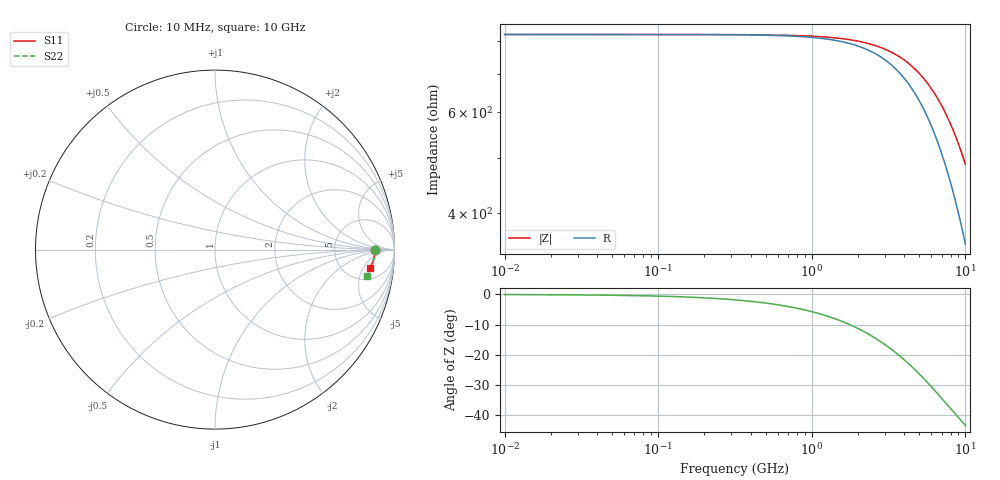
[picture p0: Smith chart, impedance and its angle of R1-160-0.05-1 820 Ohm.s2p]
!version-1
!date-03.2021
# MHz S RI R 50
!Freq ReS11 ImS11 ReS21 ImS21 ReS12 ImS12 ReS22 ImS22
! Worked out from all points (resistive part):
!   501 points, 10 MHz to 10 GHz, reference 50 ohm
!   read as one part in series: R = 820 ohm at 50 MHz
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10  0.8913 -9.71e-05  0.1087 9.47e-05  0.1087 9.47e-05  0.8913 -0.000136
430  0.8913 -0.00418  0.1088 0.00407  0.1088 0.00407  0.8912 -0.00584
850  0.8911 -0.00826  0.1089 0.00806  0.1089 0.00806  0.891 -0.0116
1270  0.8909 -0.0123  0.1092 0.012  0.1092 0.012  0.8907 -0.0173
1690  0.8906 -0.0164  0.1096 0.016  0.1096 0.016  0.8903 -0.023
2090  0.8902 -0.0203  0.11 0.0199  0.11 0.0199  0.8897 -0.0285
2510  0.8898 -0.0245  0.1106 0.0239  0.1106 0.0239  0.889 -0.0343
2930  0.8892 -0.0286  0.1113 0.028  0.1113 0.028  0.8881 -0.0401
3350  0.8885 -0.0327  0.1121 0.032  0.1121 0.032  0.8871 -0.046
3750  0.8878 -0.0367  0.113 0.0359  0.113 0.0359  0.886 -0.0516
4150  0.887 -0.0407  0.114 0.0399  0.114 0.0399  0.8848 -0.0572
4570  0.8861 -0.0449  0.1152 0.044  0.1152 0.044  0.8834 -0.0632
5010  0.885 -0.0493  0.1165 0.0484  0.1165 0.0484  0.8817 -0.0695
5410  0.8839 -0.0533  0.1179 0.0525  0.1179 0.0525  0.88 -0.0753
5810  0.8827 -0.0574  0.1194 0.0565  0.1194 0.0565  0.8782 -0.0812
6230  0.8813 -0.0617  0.1212 0.0609  0.1212 0.0609  0.876 -0.0874
6670  0.8797 -0.0663  0.1231 0.0655  0.1231 0.0655  0.8736 -0.0941
7490  0.8763 -0.0748  0.1273 0.0741  0.1273 0.0741  0.8685 -0.1066
8350  0.8722 -0.0839  0.1324 0.0835  0.1324 0.0835  0.8621 -0.1202
9170  0.8676 -0.0928  0.1381 0.0926  0.1381 0.0926  0.8551 -0.1335
9950  0.8627 -0.1013  0.1444 0.1016  0.1444 0.1016  0.8473 -0.1465
10000  0.8623 -0.1018  0.1448 0.1022  0.1448 0.1022  0.8468 -0.1473
